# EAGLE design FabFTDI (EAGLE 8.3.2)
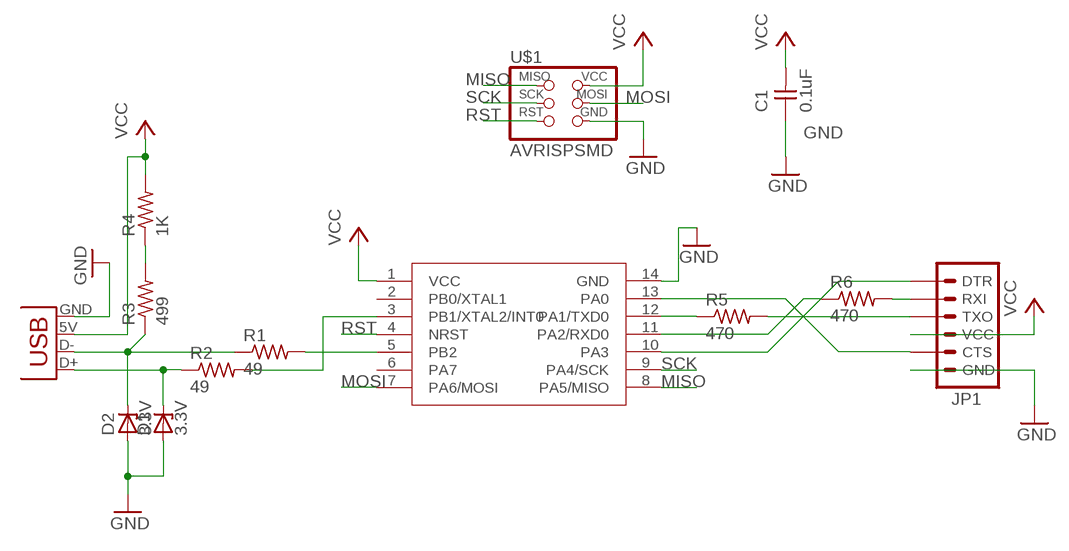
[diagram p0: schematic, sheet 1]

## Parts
C1  0.1uF  UNPOLARIZED_CAPACITOR1206  [1206]
D1  3.3V  ZENER_DIODESOD123  [SOD123]
D2  3.3V  ZENER_DIODESOD123  [SOD123]
JP1  FTDI_CONNECTORSMD  [1X06-SMD]
JP2  USBPCB  [USB_PCB]
R1  49  RESISTOR1206  [1206]
R2  49  RESISTOR1206  [1206]
R3  499  RESISTOR1206  [1206]
R4  1K  RESISTOR1206  [1206]
R5  470  RESISTOR1206  [1206]
R6  470  RESISTOR1206  [1206]
U$1  AVRISPSMD  [2X03SMD]
U$2  ATTINY441  [SOIC14]

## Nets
GND: C1.1 D1.ANODE D2.ANODE JP1.6(GND) JP2.GND U$1.6(GND) U$2.14(GND)
MISO: U$1.1(MISO) U$2.8(PA5/MISO)
MOSI: U$1.4(MOSI) U$2.7(PA6/MOSI)
N$1: D1.CATHODE JP2.D+ R2.1
N$2: D2.CATHODE JP2.D- R1.1 R3.1
N$3: R2.2 U$2.3(PB1/XTAL2/INT0)
N$4: R1.2 U$2.5(PB2)
N$5: R3.2 R4.1
N$7: JP1.2(RXI) R6.2
N$8: JP1.3(TXO) R5.2
N$9: R5.1 U$2.12(PA1/TXD0)
N$10: R6.1 U$2.11(PA2/RXD0)
N$11: JP1.5(CTS) U$2.13(PA0)
N$12: JP1.1(DTR) U$2.10(PA3)
RST: U$1.5(RST) U$2.4(NRST)
SCK: U$1.3(SCK) U$2.9(PA4/SCK)
VCC: C1.2 JP1.4(VCC) JP2.5V(VBUS) R4.2 U$1.2(VCC) U$2.1(VCC)
Unconnected: U$2.2(PB0/XTAL1) U$2.6(PA7)

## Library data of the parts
C1 = fabPatil:UNPOLARIZED_CAPACITOR: unpolarized_capacitor
D1 D2 = fabPatil:ZENER_DIODE: zener diode
JP1 = fabPatil:FTDI_CONNECTOR: FTDI connector smd
JP2 = fabPatil:USB: USB Connector Connector for USB-microB (orAB), USB-mini, and USB-PCB. For USB-micro use Digikey Part# 609-4052-1-ND (typeB) or 609-4052-1-ND (typeAB).
R1-R6 = fabPatil:RESISTOR
U$1 = fabPatil:AVRISP
U$2 = fabPatil:ATTINY441: ATTINY441

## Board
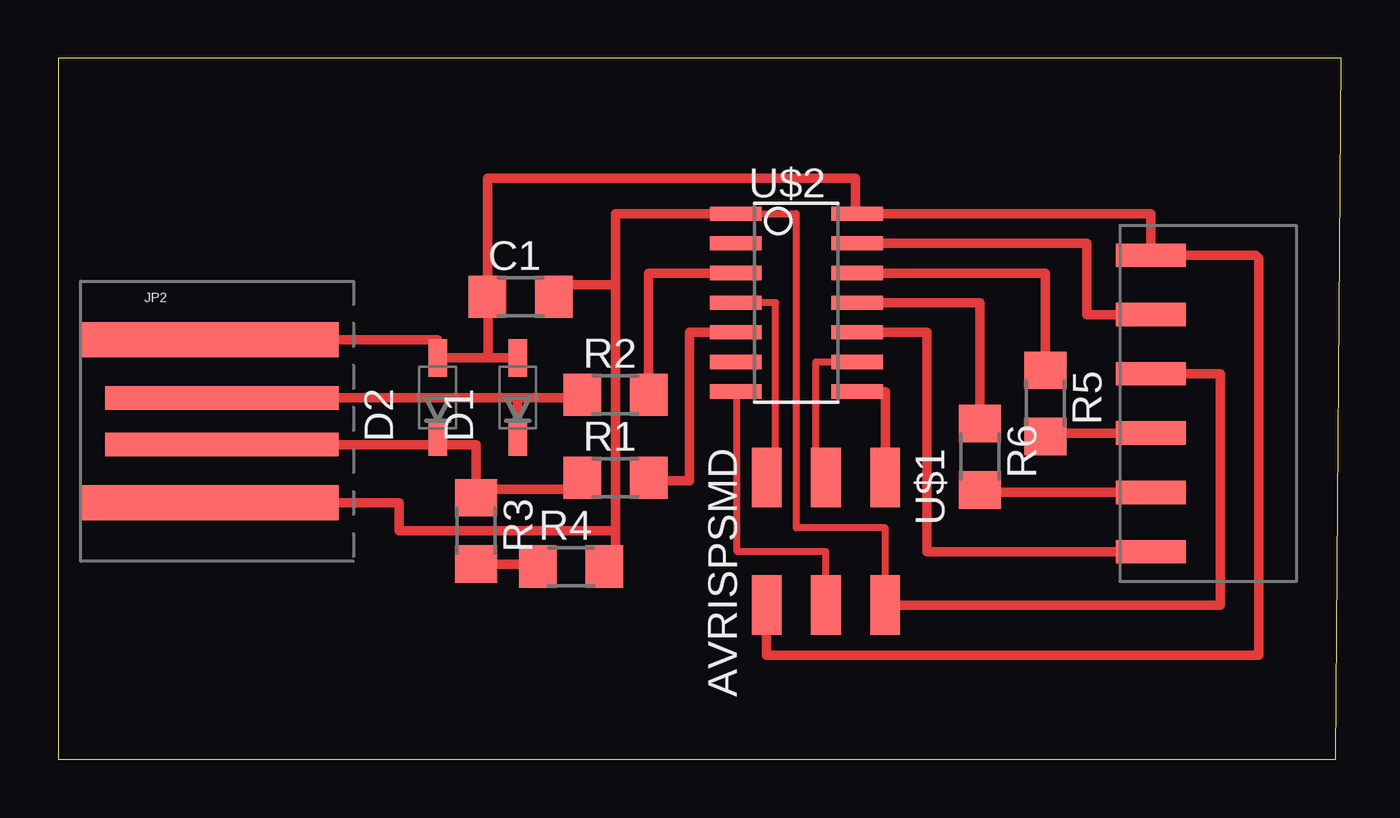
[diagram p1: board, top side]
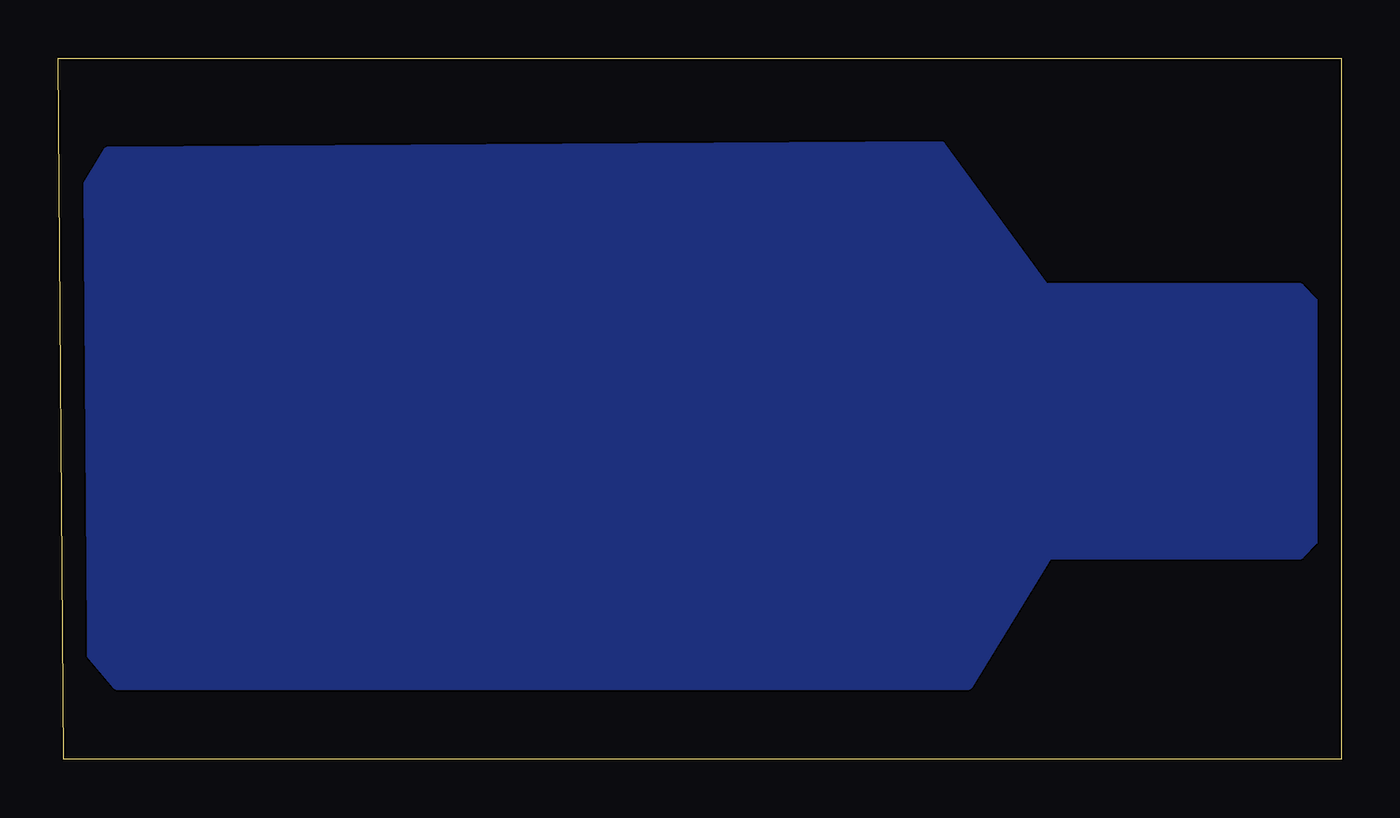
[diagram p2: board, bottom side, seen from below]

Size 54.97 x 30.02 mm. Coordinates in mm from the lower left corner, seen from the top.
Outline: 0,0 54.74,0 54.97,30.02 0,30.02 0,0
Copper layers (1*16): Top 0.035mm / dielectric 1.5mm / Bottom 0.035mm
Design rules "Patil": minimum track width 10mil, minimum drill 24mil, track to track 16mil, track to pad 16mil, pad to pad 16mil, via to via 16mil, smd to smd 16mil, copper to edge 40mil, drill to drill 8mil, minimum pad ring 10mil, minimum via ring 8mil, stop-mask expansion 4mil, vias tented up to drill 0mil, thermal gap 10mil

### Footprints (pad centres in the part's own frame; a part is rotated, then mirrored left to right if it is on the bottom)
1206 = smd 1.6 x 1.803: 1 -1.422,0; 2 1.422,0
SOD123 = smd 1.6 x 0.8: ANODE 1.7,0; CATHODE -1.7,0
1X06-SMD = smd 1 x 3: 1 -6.35,-1.35; 2 -3.81,-1.35; 3 -1.27,-1.35; 4 1.27,-1.35; 5 3.81,-1.35; 6 6.35,-1.35
USB_PCB = smd 11 x 1.5: 5V 1.55,-3.5; GND 1.55,3.5 | smd 10 x 1: D+ 2.05,1; D- 2.05,-1
2X03SMD = smd 2.54 x 1.27: 1 -2.54,2.54; 2 2.92,2.54; 3 -2.54,0; 4 2.92,0; 5 -2.54,-2.54; 6 2.92,-2.54
SOIC14 = smd 0.61 x 2.21: 1 -3.81,-2.603; 2 -2.54,-2.603; 3 -1.27,-2.603; 4 0,-2.603; 5 1.27,-2.603; 6 2.54,-2.603; 7 3.81,-2.603; 8 3.81,2.603; 9 2.54,2.603; 10 1.27,2.603; 11 0,2.603; 12 -1.27,2.603; 13 -2.54,2.603; 14 -3.81,2.603

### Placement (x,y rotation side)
C1  19.81,19.81 0 top
D1  19.68,15.49 90 top
D2  16.26,15.49 90 top
JP1  45.47,15.24 90 top
JP2  4.95,14.48 0 top
R1  23.88,12.07 0 top
R2  23.88,15.62 0 top
R3  17.91,9.78 270 top
R4  21.97,8.25 0 top
R5  42.29,15.24 270 top
R6  39.5,12.95 270 top
U$1  32.89,9.52 270 top
U$2  31.62,19.56 270 top

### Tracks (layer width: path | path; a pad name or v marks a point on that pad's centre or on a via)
GND
  Top 0.406: JP2.GND 16.26,17.98 D2.ANODE 18.41,17.19 | 18.41,17.19 D1.ANODE | 18.41,17.19 18.41,19.56 C1.1 18.39,24.89 34.16,24.89 34.16,23.37 U$2.14 46.82,23.37 JP1.6 51.31,21.59 51.44,21.46 51.44,4.45 30.35,4.45 U$1.6
MISO
  Top 0.406: U$2.8 35.43,15.75 U$1.1
MOSI
  Top 0.305: U$1.4 32.89,8.89 29.08,8.89 29.08,15.75 U$2.7
N$1
  Top 0.406: 9.55,15.24 JP2.D+ 19.68,15.48 | 19.68,15.48 D1.CATHODE | 19.68,15.48 22.45,15.48 R2.1
N$2
  Top 0.406: JP2.D- 9.33,13.46 16.26,13.46 | 16.26,13.46 D2.CATHODE | 17.91,11.56 R3.1 | 17.91,11.56 17.91,13.46 16.26,13.46 | R1.1 22.45,11.56 17.91,11.56
N$3
  Top 0.406: R2.2 25.3,20.83 U$2.3
N$4
  Top 0.406: U$2.5 27.05,18.29 27.05,11.94 25.3,11.94 R1.2
N$5
  Top 0.406: 17.91,8.25 R3.2 20.55,8.36 R4.1
N$6
  pour Bottom (no thermals): 1.14,19.56 1.78,20.19 12.7,20.19 17.14,26.29 52.83,26.04 53.85,24.38 arc-3 53.85,4.83 52.45,3.17 16,3.17 12.57,8.76 1.78,8.76 1.14,9.4
N$7
  Top 0.406: JP1.2 39.5,11.43 R6.2
N$8
  Top 0.406: JP1.3 42.29,13.97 R5.2
N$9
  Top 0.406: R5.1 42.29,20.83 U$2.12
N$10
  Top 0.406: R6.1 39.5,19.56 U$2.11
N$11
  Top 0.406: JP1.5 44.07,19.05 44.07,22.1 U$2.13
N$12
  Top 0.406: U$2.10 37.21,18.29 37.21,8.89 JP1.1
RST
  Top 0.305: U$2.4 30.73,19.56 30.73,12.45 arc-90 U$1.5
SCK
  Top 0.305: U$1.3 32.46,12.62 32.46,17.02 U$2.9
  Top 0.406: 32.64,12.19 arc90 U$1.3
VCC
  Top 0.305: U$2.1 31.62,23.37 31.62,9.91 35.43,9.91 U$1.2
  Top 0.406: 21.74,20.32 C1.2 21.23,20.32 23.88,20.32 | JP2.5V 14.61,10.98 14.61,9.78 23.88,9.78 | 23.88,20.32 23.88,9.78 | 23.88,9.78 23.88,8.25 R4.2 23.5,8.25 | U$2.1 23.88,23.37 23.88,20.32 | JP1.4 49.78,16.51 49.78,6.6 U$1.2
